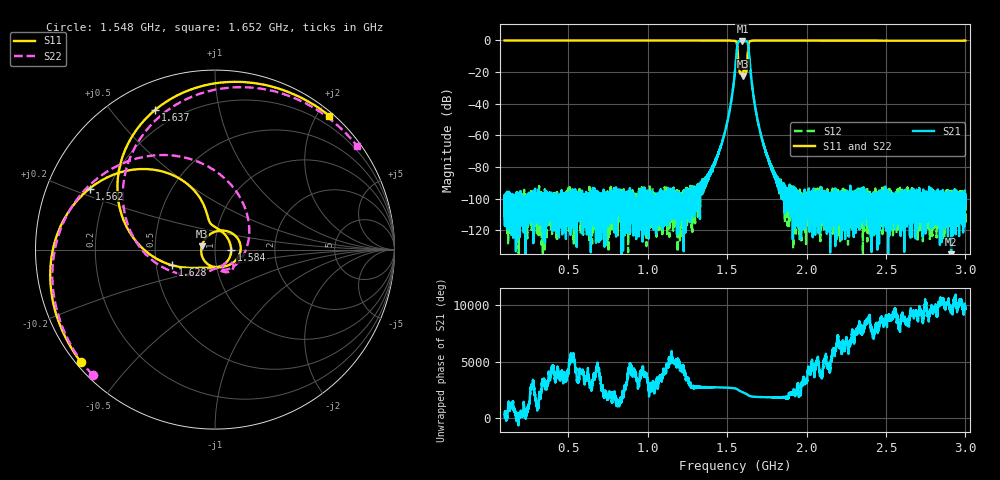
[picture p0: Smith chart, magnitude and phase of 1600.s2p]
# Hz S DB R 50
! Planar, S50180, 20087770, 20.1.2/1
! Date: 23.06.2021 14:44:44
! Data: Format (Calibration Info)
! Freq	S11:dB/Ang(F2)	S21:dB/Ang(F2)	S12:dB/Ang(F2)	S22:dB/Ang(F2)
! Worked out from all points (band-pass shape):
!   8991 points, 100 MHz to 3 GHz, reference 50 ohm
!   highest |S21| = -0.37 dB at 1.597 GHz (marker M1); lowest = -145.7 dB at 2.91 GHz (marker M2)
!   |S21| within 3 dB of the highest: 1.564 GHz to 1.633 GHz (69.09 MHz wide, 4.32 % of centre)
!   lowest |S11| = -22.4 dB at 1.597 GHz (marker M3), VSWR 1.17, Z = 43.1 + j1.68 ohm
!   |S11| at or under -10 dB: 1.569 GHz to 1.629 GHz (59.96 MHz wide, 3.75 % of centre)
!   |S22| runs from -20.5 to 0.0 dB; largest |S21 - S12| = 0.0021
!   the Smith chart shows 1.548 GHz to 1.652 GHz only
!   S11 on the Smith chart (normalised r, x): 1.548 GHz: 0.01, -0.36; 1.562 GHz: 0.13, +0.23; 1.584 GHz: 1.20, -0.01; 1.628 GHz: 0.60, -0.11; 1.637 GHz: 0.12, +0.65; 1.652 GHz: 0.05, +2.17
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1e8  0.02 154.0  -105.69 151.0  -107.20 158.1  0.01 150.1
3.119355e8  -0.03 104.2  -109.52 -19.8  -106.25 -147.0  0.00 95.5
5.835484e8  -0.01 55.1  -104.12 87.5  -103.67 11.5  0.01 45.8
1.066774e9  0.00 -6.5  -110.21 -150.0  -104.60 -108.2  0.04 -12.3
1.410645e9  -0.01 -52.8  -79.53 -142.1  -80.82 -144.6  0.03 -53.6
1.495161e9  -0.04 -79.7  -54.40 -169.5  -54.35 -170.2  -0.00 -77.4
1.548387e9  -0.22 -140.0  -21.04 130.2  -21.04 130.1  -0.21 -134.3
1.55e9  -0.26 -144.6  -19.42 125.4  -19.41 125.3  -0.25 -139.1
1.562258e9  -2.19 154.0  -5.41 57.5  -5.41 57.4  -2.33 148.6
1.583548e9  -20.93 -2.5  -0.41 -126.8  -0.41 -126.9  -20.16 -70.7
1.596774e9  -22.33 176.6  -0.37 150.5  -0.38 150.4  -20.49 -53.2
1.597419e9  -22.35 165.3  -0.37 146.6  -0.38 146.5  -20.47 -51.0
1.614839e9  -17.87 -30.7  -0.43 38.5  -0.44 38.5  -17.66 -70.1
1.627742e9  -11.85 -160.1  -0.85 -61.3  -0.86 -61.4  -11.90 -149.5
1.637419e9  -1.45 113.2  -7.34 -158.2  -7.34 -158.3  -1.48 103.3
1.651935e9  -0.17 49.5  -23.34 135.2  -23.35 135.0  -0.18 36.0
1.70129e9  -0.04 -6.3  -54.71 79.9  -54.67 79.8  0.01 -15.8
1.776452e9  -0.01 -31.5  -78.59 56.1  -79.32 57.8  -0.02 -38.4
2.033548e9  -0.04 -65.4  -103.36 11.6  -96.51 82.5  -0.01 -68.3
2.516774e9  -0.07 -104.6  -108.91 120.1  -106.14 -15.2  -0.05 -104.0
2.910323e9  -0.14 -133.5  -145.72 65.1  -103.93 100.0  -0.12 -130.5
3e9  -0.10 -140.1  -100.97 70.1  -102.36 -109.8  -0.09 -137.0
